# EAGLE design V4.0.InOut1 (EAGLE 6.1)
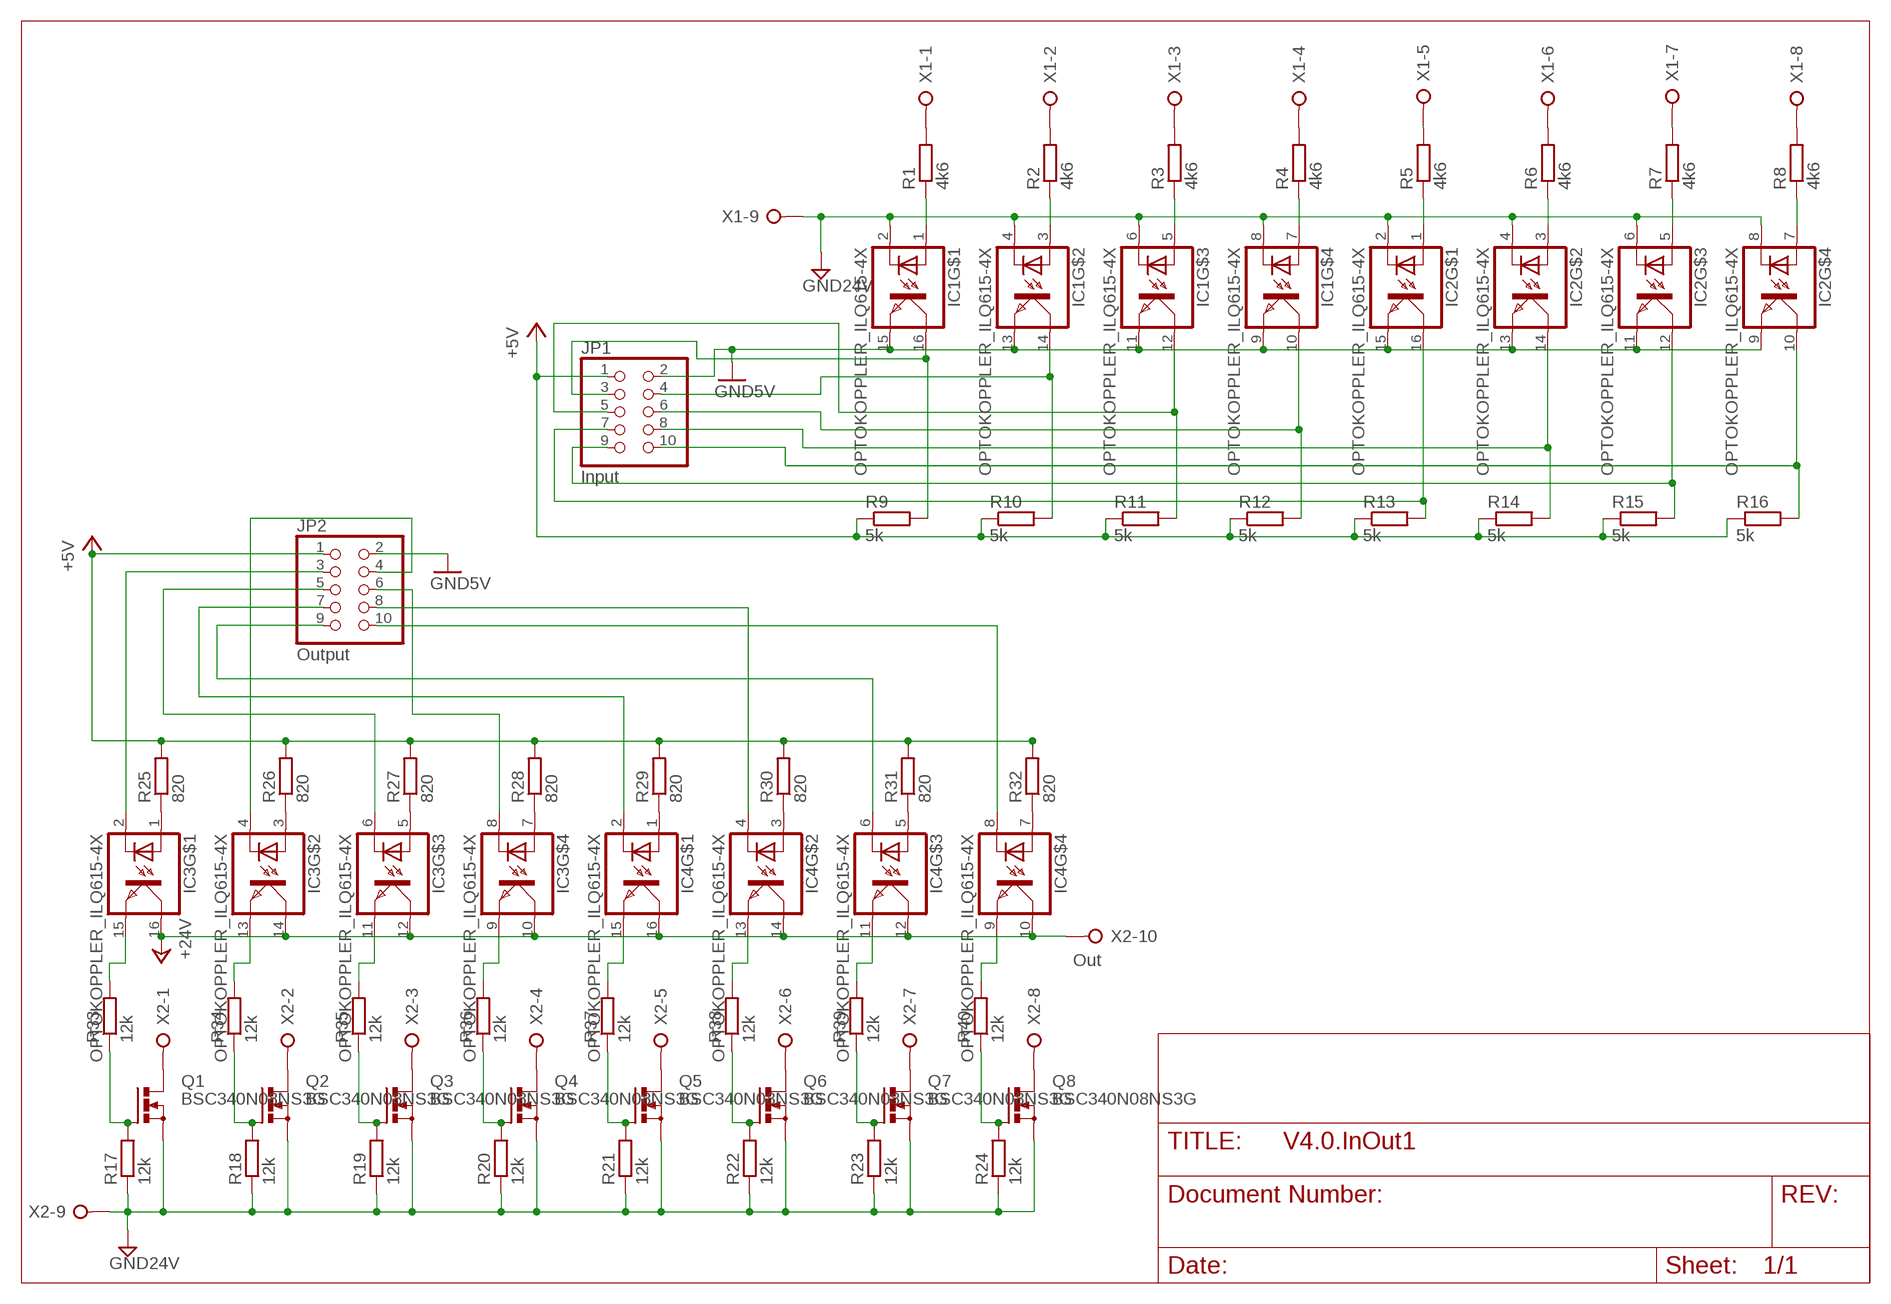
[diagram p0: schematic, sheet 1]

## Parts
IC1  OPTOKOPPLER_ILQ615-4X  [OPTOKOPPLER_ILQ615-4X]
IC2  OPTOKOPPLER_ILQ615-4X  [OPTOKOPPLER_ILQ615-4X]
IC3  OPTOKOPPLER_ILQ615-4X  [OPTOKOPPLER_ILQ615-4X]
IC4  OPTOKOPPLER_ILQ615-4X  [OPTOKOPPLER_ILQ615-4X]
JP1  Input  PINHD-2X5  [2X05]
JP2  Output  PINHD-2X5  [2X05]
Q1  BSC340N08NS3G  [PG-TDSON-8]
Q2  BSC340N08NS3G  [PG-TDSON-8]
Q3  BSC340N08NS3G  [PG-TDSON-8]
Q4  BSC340N08NS3G  [PG-TDSON-8]
Q5  BSC340N08NS3G  [PG-TDSON-8]
Q6  BSC340N08NS3G  [PG-TDSON-8]
Q7  BSC340N08NS3G  [PG-TDSON-8]
Q8  BSC340N08NS3G  [PG-TDSON-8]
R1  4k6  R-EU_R1206  [R1206]
R2  4k6  R-EU_R1206  [R1206]
R3  4k6  R-EU_R1206  [R1206]
R4  4k6  R-EU_R1206  [R1206]
R5  4k6  R-EU_R1206  [R1206]
R6  4k6  R-EU_R1206  [R1206]
R7  4k6  R-EU_R1206  [R1206]
R8  4k6  R-EU_R1206  [R1206]
R9  5k  R-EU_R0402  [R0402]
R10  5k  R-EU_R0402  [R0402]
R11  5k  R-EU_R0402  [R0402]
R12  5k  R-EU_R0402  [R0402]
R13  5k  R-EU_R0402  [R0402]
R14  5k  R-EU_R0402  [R0402]
R15  5k  R-EU_R0402  [R0402]
R16  5k  R-EU_R0402  [R0402]
R17  12k  R-EU_R0402  [R0402]
R18  12k  R-EU_R0402  [R0402]
R19  12k  R-EU_R0402  [R0402]
R20  12k  R-EU_R0402  [R0402]
R21  12k  R-EU_R0402  [R0402]
R22  12k  R-EU_R0402  [R0402]
R23  12k  R-EU_R0402  [R0402]
R24  12k  R-EU_R0402  [R0402]
R25  820  R-EU_R0402  [R0402]
R26  820  R-EU_R0402  [R0402]
R27  820  R-EU_R0402  [R0402]
R28  820  R-EU_R0402  [R0402]
R29  820  R-EU_R0402  [R0402]
R30  820  R-EU_R0402  [R0402]
R31  820  R-EU_R0402  [R0402]
R32  820  R-EU_R0402  [R0402]
R33  12k  R-EU_R0402  [R0402]
R34  12k  R-EU_R0402  [R0402]
R35  12k  R-EU_R0402  [R0402]
R36  12k  R-EU_R0402  [R0402]
R37  12k  R-EU_R0402  [R0402]
R38  12k  R-EU_R0402  [R0402]
R39  12k  R-EU_R0402  [R0402]
R40  12k  R-EU_R0402  [R0402]
X1  In  W237-10P  [W237-10P]
X2  Out  W237-10P  [W237-10P]

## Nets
+5V_IN [+5V]: JP1.1 R9.1 R10.1 R11.1 R12.1 R13.1 R14.1 R15.1 R16.1 ; supply symbol labelled +5V
+5V_OUT [+5V]: JP2.1 R25.2 R26.2 R27.2 R28.2 R29.2 R30.2 R31.2 R32.2 ; supply symbol labelled +5V
+24V: IC3.10(COL) IC3.12(COL) IC3.14(COL) IC3.16(COL) IC4.10(COL) IC4.12(COL) IC4.14(COL) IC4.16(COL) X2.10
AGND_IN [+24V]: IC1.2(C) IC1.4(C) IC1.6(C) IC1.8(C) IC2.2(C) IC2.4(C) IC2.6(C) IC2.8(C) X1.9 ; supply symbol labelled GND24V
AGND_OUT [+24V]: Q1.1(S) Q1.2(S) Q1.3(S) Q2.1(S) Q2.2(S) Q2.3(S) Q3.1(S) Q3.2(S) Q3.3(S) Q4.1(S) Q4.2(S) Q4.3(S) Q5.1(S) Q5.2(S) Q5.3(S) Q6.1(S) Q6.2(S) Q6.3(S) Q7.1(S) Q7.2(S) Q7.3(S) Q8.1(S) Q8.2(S) Q8.3(S) R17.1 R18.1 R19.1 R20.1 R21.1 R22.1 R23.1 R24.1 X2.9 ; supply symbol labelled GND24V
GND [+5V GND]: IC1.9(EMIT) IC1.11(EMIT) IC1.13(EMIT) IC1.15(EMIT) IC2.9(EMIT) IC2.11(EMIT) IC2.13(EMIT) IC2.15(EMIT) JP1.2 JP2.2 ; supply symbol labelled GND5V
N$1: R1.2 X1.1
N$2: R2.2 X1.2
N$3: R3.2 X1.3
N$4: R4.2 X1.4
N$5: R5.2 X1.5
N$6: R6.2 X1.6
N$7: R7.2 X1.7
N$8: R8.2 X1.8
N$9: IC1.16(COL) JP1.3 R9.2
N$10: IC1.1(A) R1.1
N$11: IC1.3(A) R2.1
N$12: IC1.5(A) R3.1
N$13: IC1.7(A) R4.1
N$14: IC2.1(A) R5.1
N$15: IC2.3(A) R6.1
N$16: IC2.5(A) R7.1
N$17: IC2.7(A) R8.1
N$18: IC1.14(COL) JP1.4 R10.2
N$19: IC1.12(COL) JP1.5 R11.2
N$20: IC1.10(COL) JP1.6 R12.2
N$21: IC2.16(COL) JP1.7 R13.2
N$22: IC2.14(COL) JP1.8 R14.2
N$23: IC2.12(COL) JP1.9 R15.2
N$24: IC2.10(COL) JP1.10 R16.2
N$25: Q1.4(G) R17.2 R33.1
N$26: Q2.4(G) R18.2 R34.1
N$27: Q3.4(G) R19.2 R35.1
N$28: Q4.4(G) R20.2 R36.1
N$29: Q5.4(G) R21.2 R37.1
N$30: Q6.4(G) R22.2 R38.1
N$31: Q7.4(G) R23.2 R39.1
N$32: Q8.4(G) R24.2 R40.1
N$33: IC3.3(A) R26.1
N$34: Q1.5(D) Q1.6(D) Q1.7(D) Q1.8(D) X2.1
N$35: IC3.5(A) R27.1
N$36: Q2.5(D) Q2.6(D) Q2.7(D) Q2.8(D) X2.2
N$37: Q3.5(D) Q3.6(D) Q3.7(D) Q3.8(D) X2.3
N$38: Q4.5(D) Q4.6(D) Q4.7(D) Q4.8(D) X2.4
N$39: Q5.5(D) Q5.6(D) Q5.7(D) Q5.8(D) X2.5
N$40: Q6.5(D) Q6.6(D) Q6.7(D) Q6.8(D) X2.6
N$41: Q7.5(D) Q7.6(D) Q7.7(D) Q7.8(D) X2.7
N$42: Q8.5(D) Q8.6(D) Q8.7(D) Q8.8(D) X2.8
N$43: IC3.7(A) R28.1
N$44: IC3.1(A) R25.1
N$45: IC4.1(A) R29.1
N$46: IC4.3(A) R30.1
N$47: IC4.5(A) R31.1
N$48: IC4.7(A) R32.1
N$49: IC3.15(EMIT) R33.2
N$50: IC3.2(C) JP2.3
N$51: IC3.4(C) JP2.4
N$52: IC3.6(C) JP2.5
N$53: IC3.8(C) JP2.6
N$54: IC4.2(C) JP2.7
N$55: IC4.4(C) JP2.8
N$56: IC4.6(C) JP2.9
N$57: IC4.8(C) JP2.10
N$58: IC3.13(EMIT) R34.2
N$59: IC3.11(EMIT) R35.2
N$60: IC3.9(EMIT) R36.2
N$61: IC4.15(EMIT) R37.2
N$62: IC4.13(EMIT) R38.2
N$63: IC4.11(EMIT) R39.2
N$64: IC4.9(EMIT) R40.2
Unconnected: Q1.TH Q2.TH Q3.TH Q4.TH Q5.TH Q6.TH Q7.TH Q8.TH X1.10

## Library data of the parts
IC1-IC4 = Jonas_Bib_Eagle:OPTOKOPPLER_ILQ615-4X: ILQ615-4X009
JP1 JP2 = pinhead:PINHD-2X5: PIN HEADER
Q1-Q8 = transistor-power:BSC340N08NS3G: OptiMOS TM 3 Power-Transistor BSC340N08NS3 G Source: Data sheet
R1-R40 = rcl:R-EU_: RESISTOR, European symbol
X1 X2 = con-wago-508:W237-10P: WAGO SREW CLAMP; OC_FARNELL: unknown; OC_NEWARK: unknown

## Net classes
0 default: width 0.305 mm
1 +5V: width 0.508 mm
2 +5V GND: width 0.508 mm
3 +24V: width 0.508 mm
4 +24V GND: width 0.508 mm

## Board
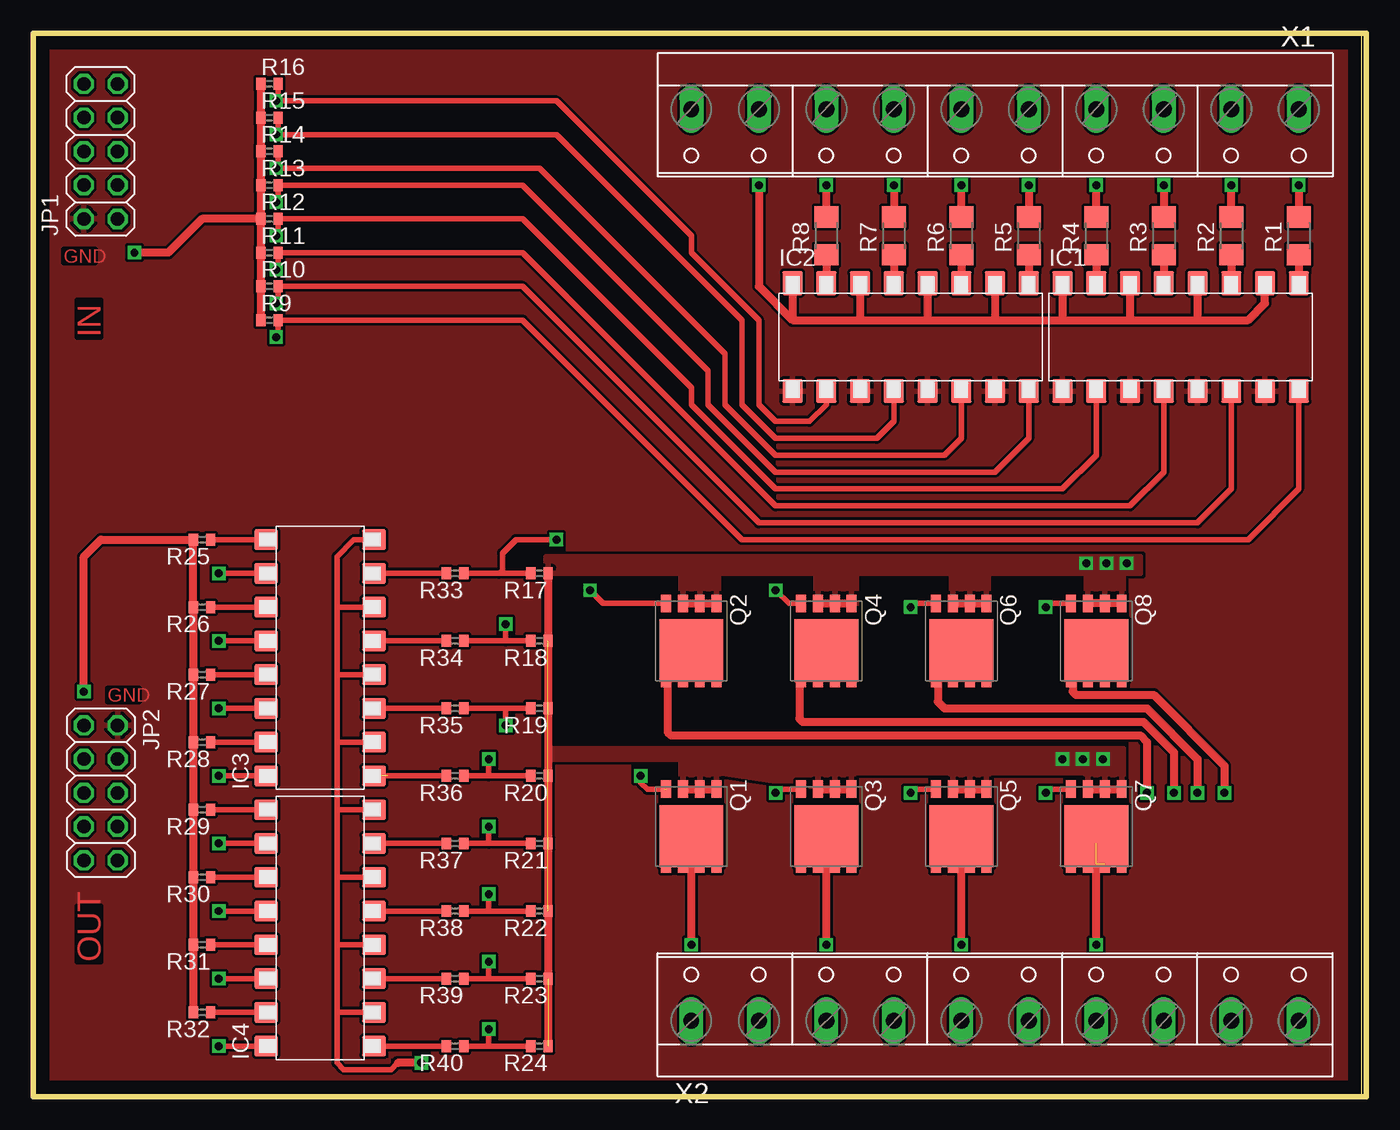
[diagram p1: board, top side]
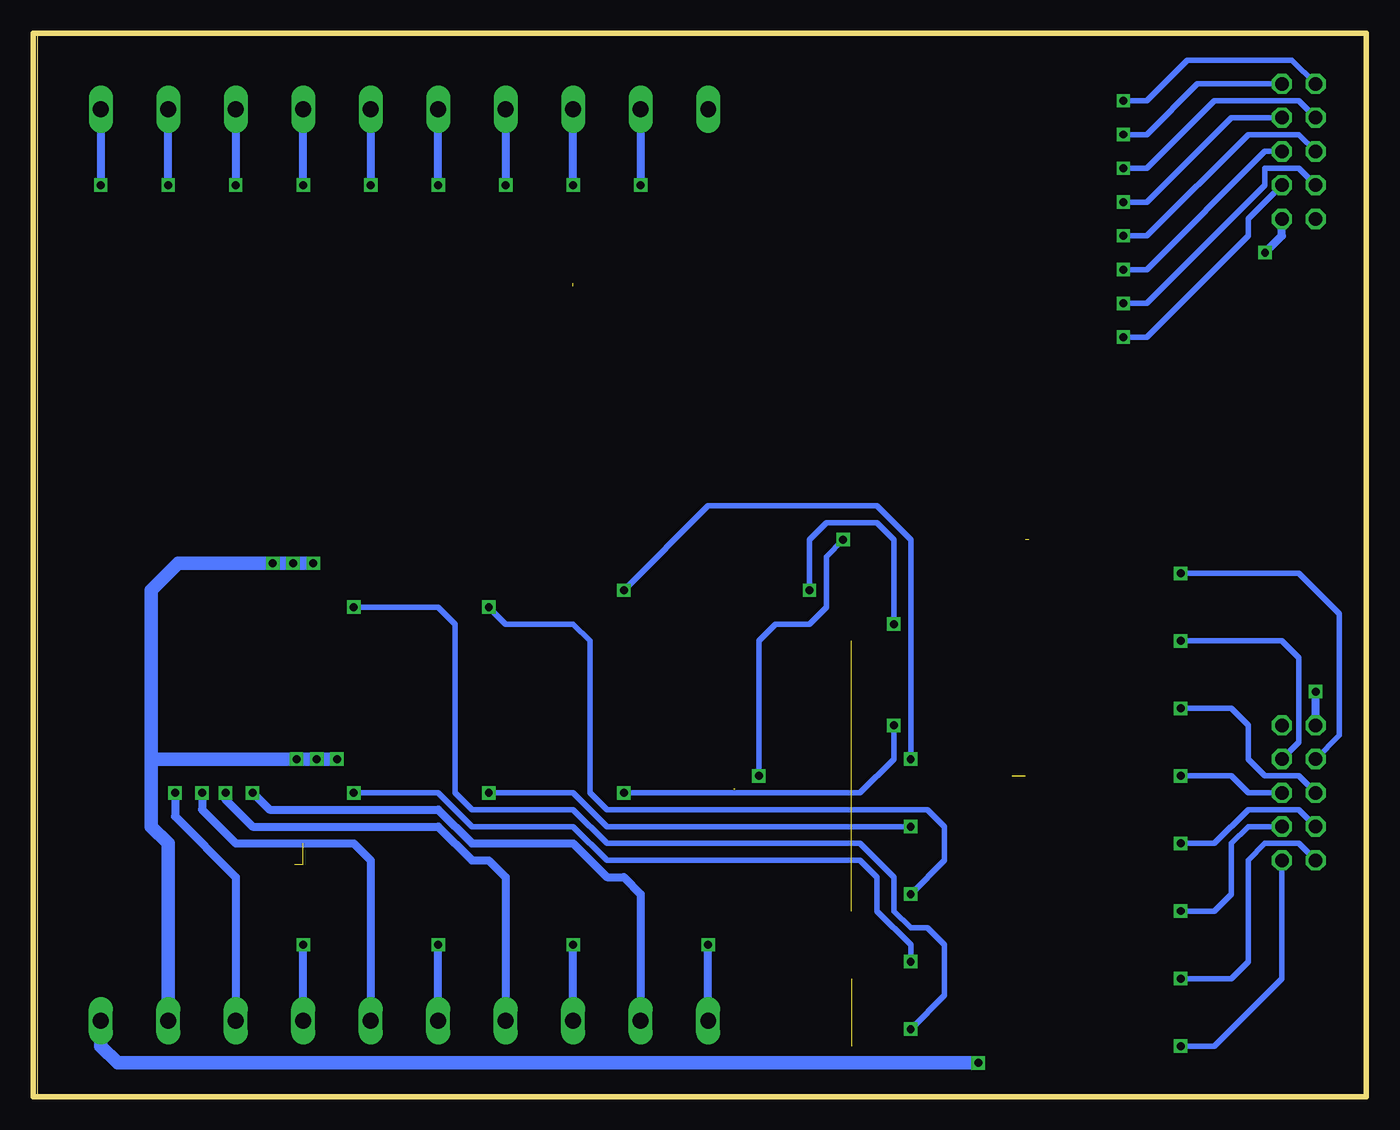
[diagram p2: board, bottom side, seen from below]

Size 100.33 x 80.01 mm. Coordinates in mm from the lower left corner, seen from the top.
Outline: 0,0 100,0 100,80 0,80
Outline: 0,0 100.33,0 100.33,80.01 0,80.01 0,0
Copper layers (1*16): Top 0.035mm / dielectric 1.5mm / Bottom 0.035mm
Design rules: minimum track width 10mil, minimum drill 24mil, track to track 8mil, track to pad 8mil, pad to pad 8mil, via to via 8mil, smd to smd 8mil, copper to edge 40mil, drill to drill 8mil, minimum pad ring 10mil, minimum via ring 8mil, stop-mask expansion 4mil, vias tented up to drill 0mil, thermal gap 10mil

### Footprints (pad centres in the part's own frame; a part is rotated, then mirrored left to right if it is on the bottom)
OPTOKOPPLER_ILQ615-4X = smd 1.525 x 1.78: 1 8.89,4.06; 2 6.35,4.06; 3 3.81,4.06; 4 1.27,4.06; 5 -1.27,4.06; 6 -3.81,4.06; 7 -6.35,4.06; 8 -8.89,4.06; 9 -8.89,-4.06; 10 -6.35,-4.06; 11 -3.81,-4.06; 12 -1.27,-4.06; 13 1.27,-4.06; 14 3.81,-4.06; 15 6.35,-4.06; 16 8.89,-4.06
2X05 = drill 1.016 octagon: 1 -5.08,-1.27; 2 -5.08,1.27; 3 -2.54,-1.27; 4 -2.54,1.27; 5 0,-1.27; 6 0,1.27; 7 2.54,-1.27; 8 2.54,1.27; 9 5.08,-1.27; 10 5.08,1.27
PG-TDSON-8 = smd 1.3 x 0.75: 1 -2.825,1.905; 2 -2.825,0.635; 3 -2.825,-0.635; 4 -2.825,-1.905; 5 2.825,-1.905; 6 2.825,-0.635; 7 2.825,0.635; 8 2.825,1.905 | smd 4.7 x 4.8: TH 0.725,0
R1206 = smd 1.6 x 1.803: 1 -1.422,0; 2 1.422,0
R0402 = smd 0.7 x 0.9: 1 -0.65,0; 2 0.65,0
W237-10P = drill 1.194 long: 1 -22.86,-0.635; 2 -17.78,-0.635; 3 -12.7,-0.635; 4 -7.62,-0.635; 5 -2.54,-0.635; 6 2.54,-0.635; 7 7.62,-0.635; 8 12.7,-0.635; 9 17.78,-0.635; 10 22.86,-0.635

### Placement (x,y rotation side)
IC1  86.36,57.15 0 top
IC2  66.04,57.15 0 top
IC3  21.59,33.02 90 top
IC4  21.59,12.7 90 top
JP1  5.08,71.12 90 top
JP2  5.08,22.86 270 top
Q1  49.53,20.32 270 top
Q2  49.53,34.29 270 top
Q3  59.69,20.32 270 top
Q4  59.69,34.29 270 top
Q5  69.85,20.32 270 top
Q6  69.85,34.29 270 top
Q7  80.01,20.32 270 top
Q8  80.01,34.29 270 top
R1  95.25,64.77 90 top
R2  90.17,64.77 90 top
R3  85.09,64.77 90 top
R4  80.01,64.77 90 top
R5  74.93,64.77 90 top
R6  69.85,64.77 90 top
R7  64.77,64.77 90 top
R8  59.69,64.77 90 top
R9  17.78,58.42 0 top
R10  17.78,60.96 0 top
R11  17.78,63.5 0 top
R12  17.78,66.04 0 top
R13  17.78,68.58 0 top
R14  17.78,71.12 0 top
R15  17.78,73.66 0 top
R16  17.78,76.2 0 top
R17  38.1,39.37 180 top
R18  38.1,34.29 180 top
R19  38.1,29.21 180 top
R20  38.1,24.13 180 top
R21  38.1,19.05 180 top
R22  38.1,13.97 180 top
R23  38.1,8.89 180 top
R24  38.1,3.81 180 top
R25  12.7,41.91 180 top
R26  12.7,36.83 180 top
R27  12.7,31.75 180 top
R28  12.7,26.67 180 top
R29  12.7,21.59 180 top
R30  12.7,16.51 180 top
R31  12.7,11.43 180 top
R32  12.7,6.35 180 top
R33  31.75,39.37 180 top
R34  31.75,34.29 180 top
R35  31.75,29.21 180 top
R36  31.75,24.13 180 top
R37  31.75,19.05 180 top
R38  31.75,13.97 180 top
R39  31.75,8.89 180 top
R40  31.75,3.81 180 top
X1  72.39,73.66 180 top
X2  72.39,6.35 0 top

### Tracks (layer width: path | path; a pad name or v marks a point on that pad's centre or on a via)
+5V_IN  (via drill 0.6)
  Top 0.61: R12.1 12.7,66.04 10.16,63.5 v7.62,63.5 | R16.1 R15.1 R14.1 R13.1 R12.1 | R12.1 R11.1 R10.1 R9.1
  Bottom 0.61: v7.62,63.5 6.35,64.77 JP1.1
+5V_OUT  (via drill 0.6)
  Top 0.61: v3.81,30.48 3.81,40.64 5.08,41.91 R25.2 R26.2 R27.2 R28.2 R29.2 R30.2 R31.2 R32.2
  Bottom 0.61: JP2.1 v3.81,30.48
+24V  (via drill 0.6)  (1 unrouted)
  Top 0.406: 27.43,2.54 26.92,2.03 23.37,2.03 22.86,2.54 22.86,6.35 | 22.86,6.35 22.86,11.43 | 22.86,11.43 22.86,16.51 | 22.86,16.51 22.86,21.59 | 22.86,21.59 22.86,26.67 | 22.86,26.67 22.86,31.75 | 22.86,31.75 22.86,36.83 | 22.86,36.83 22.86,40.64 24.13,41.91 25.4,41.91 | IC3.14 22.86,36.83 | IC3.12 22.86,31.75 | IC3.10 22.86,26.67 | IC4.10 22.86,6.35 | IC4.12 22.86,11.43 | IC4.14 22.86,16.51 | IC4.16 22.86,21.59
  Top 0.61: v29.21,2.54 27.43,2.54
  Bottom 1.016: X2.10 95.25,3.81 93.98,2.54 v29.21,2.54
AGND_IN  (via drill 0.6)
  Top 0.61: v54.61,68.58 54.61,60.96 57.15,58.42 | 57.15,58.42 62.23,58.42 | 62.23,58.42 67.31,58.42 | 67.31,58.42 72.39,58.42 | 72.39,58.42 77.47,58.42 | 77.47,58.42 82.55,58.42 | 82.55,58.42 87.63,58.42 | 87.63,58.42 91.44,58.42 92.71,59.69 IC1.2 | IC2.8 57.15,58.42 | IC2.6 62.23,58.42 | IC2.4 67.31,58.42 | IC2.2 72.39,58.42 | IC1.8 77.47,58.42 | IC1.6 82.55,58.42 | IC1.4 87.63,58.42
  Bottom 0.61: X1.9 v54.61,68.58
AGND_OUT  (via drill 0.6)  (6 unrouted)
  Top 0.406: 79.53,37.12 79.5,37.08
  Top 0.61: R20.1 R24.1 | Q2.3 Q2.1 | Q4.3 Q4.1 | Q6.3 Q6.1 | Q1.3 51.28,23.14 | Q3.3 Q3.1 | Q5.3 Q5.1 | Q7.3 Q7.1 | Q8.1 79.53,37.12 | R17.1 38.75,24.24
  Bottom 1.016: X2.9 90.17,19.05 91.44,20.32 91.44,25.4 | 91.44,25.4 91.44,38.1 89.41,40.13 v82.3,40.13 v80.77,40.13 v79.25,40.13 | 91.44,25.4 v80.52,25.4 v78.99,25.4 v77.47,25.4
  pour Top: 82.55,40.64 38.61,40.64 38.61,39.37 48.77,39.37 48.77,36.83 51.56,36.83 51.56,38.86 51.56,39.37 58.93,39.37 58.93,36.83 61.98,36.83 61.98,39.37 69.09,39.37 69.09,37.08 71.88,37.08 71.88,39.37 79.25,39.37 79.25,36.83 82.04,36.83 82.04,39.37 82.55,39.37 83.31,39.37 83.31,40.64
  pour Top: 38.86,25.4 48.77,25.4 48.77,22.86 51.56,22.86 51.56,24.38 61.72,22.86 61.72,24.38 69.09,24.38 69.09,22.86 71.88,22.86 71.88,24.38 79.25,24.38 79.25,22.86 82.04,22.86 82.04,26.16 38.86,26.16
GND
  pour Top (rank 2): 0,80.01 0,0 100.33,0 100.33,80.01
N$1  (via drill 0.6)
  Top 0.61: v95.25,68.58 R1.2
  Bottom 0.61: X1.1 v95.25,68.58
N$2  (via drill 0.6)
  Top 0.61: R2.2 v90.17,68.58
  Bottom 0.61: v90.17,68.58 X1.2
N$3  (via drill 0.6)
  Top 0.61: v85.09,68.58 R3.2
  Bottom 0.61: X1.3 v85.09,68.58
N$4  (via drill 0.6)
  Top 0.61: R4.2 v80.01,68.58
  Bottom 0.61: v80.01,68.58 X1.4
N$5  (via drill 0.6)
  Top 0.61: v74.93,68.58 R5.2
  Bottom 0.61: X1.5 v74.93,68.58
N$6  (via drill 0.6)
  Top 0.61: R6.2 v69.85,68.58
  Bottom 0.61: v69.85,68.58 X1.6
N$7  (via drill 0.6)
  Top 0.61: v64.77,68.58 R7.2
  Bottom 0.61: X1.7 v64.77,68.58
N$8  (via drill 0.6)
  Top 0.61: R8.2 v59.69,68.58
  Bottom 0.61: v59.69,68.58 X1.8
N$9  (via drill 0.6)
  Top 0.406: IC1.16 95.25,45.72 91.44,41.91 53.34,41.91 36.83,58.42 R9.2 18.43,57.29 v18.29,57.15
  Bottom 0.406: v18.29,57.15 16.51,57.15 8.89,64.77 8.89,66.04 JP1.3
N$10
  Top 0.61: R1.1 IC1.1
N$11
  Top 0.61: R2.1 IC1.3
N$12
  Top 0.61: R3.1 IC1.5
N$13
  Top 0.61: R4.1 IC1.7
N$14
  Top 0.61: R5.1 IC2.1
N$15
  Top 0.61: R6.1 IC2.3
N$16
  Top 0.61: R7.1 IC2.5
N$17  (1 unrouted)
  Top 0.61: R8.1 59.69,60.96
N$18  (via drill 0.6)
  Top 0.406: IC1.14 90.17,45.72 87.63,43.18 54.61,43.18 36.83,60.96 R10.2 18.43,59.83 v18.29,59.69
  Bottom 0.406: v18.29,59.69 16.51,59.69 7.62,68.58 7.62,69.85 5.08,69.85 JP1.4
N$19  (via drill 0.6)
  Top 0.406: IC1.12 85.09,46.99 82.55,44.45 55.88,44.45 36.83,63.5 R11.2 18.43,62.37 v18.29,62.23
  Bottom 0.406: v18.29,62.23 16.51,62.23 7.62,71.12 JP1.5
N$20  (via drill 0.6)
  Top 0.406: IC1.10 80.01,48.26 77.47,45.72 55.88,45.72 49.53,52.07 49.53,53.34 36.83,66.04 R12.2 18.43,64.91 v18.29,64.77
  Bottom 0.406: v18.29,64.77 16.51,64.77 8.89,72.39 5.08,72.39 JP1.6
N$21  (via drill 0.6)
  Top 0.406: IC2.16 74.93,49.53 72.39,46.99 55.88,46.99 50.8,52.07 50.8,54.61 36.83,68.58 R13.2 18.43,67.45 v18.29,67.31
  Bottom 0.406: v18.29,67.31 16.51,67.31 10.16,73.66 JP1.7
N$22  (via drill 0.6)
  Top 0.406: R14.2 18.43,69.99 v18.29,69.85 38.1,69.85 52.07,55.88 52.07,52.07 55.88,48.26 68.58,48.26 69.85,49.53 IC2.14
  Bottom 0.406: v18.29,69.85 16.51,69.85 11.43,74.93 5.08,74.93 JP1.8
N$23  (via drill 0.6)
  Top 0.406: R15.2 18.43,72.53 v18.29,72.39 39.37,72.39 53.34,58.42 53.34,52.07 55.88,49.53 63.5,49.53 64.77,50.8 IC2.12
  Bottom 0.406: v18.29,72.39 16.51,72.39 12.7,76.2 JP1.9
N$24  (via drill 0.6)
  Top 0.406: R16.2 18.43,75.07 v18.29,74.93 39.37,74.93 49.53,64.77 49.53,63.5 54.61,58.42 54.61,52.07 55.88,50.8 58.42,50.8 59.69,52.07 IC2.10
  Bottom 0.406: v18.29,74.93 16.51,74.93 13.46,77.98 5.59,77.98 JP1.10
N$25  (via drill 0.6)  (1 unrouted)
  Top 0.406: R17.2 35.05,39.37 | 35.05,39.37 R33.1 | v39.37,41.91 36.32,41.91 35.31,40.89 35.31,39.62 35.05,39.37 | v45.72,24.13 45.72,23.62 46.23,23.11 47.5,23.11
  Bottom 0.406: v39.37,41.91 40.64,40.64 40.64,36.83 41.91,35.56 44.45,35.56 45.72,34.29 v45.72,24.13
N$26  (via drill 0.6)
  Top 0.406: R18.2 35.56,34.29 | 35.56,34.29 R34.1 | Q2.4 42.9,37.12 v41.91,38.1 | v35.56,35.56 35.56,34.29
  Bottom 0.406: v41.91,38.1 41.91,41.91 40.64,43.18 36.83,43.18 35.56,41.91 v35.56,35.56
N$27  (via drill 0.6)
  Top 0.406: R19.2 35.56,29.21 | 35.56,29.21 R35.1 | Q3.4 56.16,23.14 v55.88,22.86 | v35.56,27.94 35.56,29.21
  Bottom 0.406: v55.88,22.86 38.1,22.86 35.56,25.4 v35.56,27.94
N$28  (via drill 0.6)
  Top 0.406: R20.2 34.29,24.13 | 34.29,24.13 R36.1 | Q4.4 56.87,37.12 v55.88,38.1 | v34.29,25.4 34.29,24.13
  Bottom 0.406: v55.88,38.1 49.53,44.45 36.83,44.45 34.29,41.91 v34.29,25.4
N$29  (via drill 0.6)
  Top 0.406: R21.2 34.29,19.05 | 34.29,19.05 R37.1 | Q5.4 66.33,23.14 v66.04,22.86 | v34.29,20.32 34.29,19.05
  Bottom 0.406: v66.04,22.86 59.69,22.86 57.15,20.32 v34.29,20.32
N$30  (via drill 0.6)
  Top 0.406: R22.2 34.29,13.97 | 34.29,13.97 R38.1 | Q6.4 66.33,37.12 v66.04,36.83 | v34.29,15.24 34.29,13.97
  Bottom 0.406: v66.04,36.83 64.77,35.56 59.69,35.56 58.42,34.29 58.42,22.86 57.15,21.59 33.02,21.59 31.75,20.32 31.75,17.78 v34.29,15.24
N$31  (via drill 0.6)
  Top 0.406: R23.2 34.29,8.89 | 34.29,8.89 R39.1 | Q7.4 76.48,23.14 v76.2,22.86 | v34.29,10.16 34.29,8.89
  Bottom 0.406: v76.2,22.86 69.85,22.86 67.31,20.32 59.69,20.32 57.15,17.78 38.1,17.78 36.83,16.51 36.83,13.97 34.29,11.43 v34.29,10.16
N$32  (via drill 0.6)
  Top 0.406: R24.2 34.29,3.81 | 34.29,3.81 R40.1 | Q8.4 76.48,37.12 v76.2,36.83 | v34.29,5.08 34.29,3.81
  Bottom 0.406: v76.2,36.83 69.85,36.83 68.58,35.56 68.58,22.86 67.31,21.59 59.69,21.59 57.15,19.05 38.1,19.05 35.56,16.51 35.56,13.97 34.29,12.7 33.02,12.7 31.75,11.43 31.75,7.62 v34.29,5.08
N$33
  Top 0.406: R26.1 IC3.3
N$34  (via drill 0.6)
  Top 0.61: v49.53,11.43 49.53,17.5 | 49.53,19.05 49.53,17.78 49.53,17.5 | Q1.7 49.53,17.5
  Bottom 0.61: X2.1 v49.53,11.43
N$35
  Top 0.406: R27.1 IC3.5
N$36  (via drill 0.6)
  Top 0.406: Q2.8 47.98,31.46 47.75,31.24
  Top 0.61: 47.75,31.24 47.75,27.43 48.01,27.18 83.31,27.18 83.82,26.67 v83.82,22.86
  Bottom 0.61: v83.82,22.86 82.55,21.59 69.85,21.59 67.31,19.05 59.69,19.05 57.15,16.51 55.88,16.51 54.61,15.24 X2.2
N$37  (via drill 0.6)
  Top 0.61: v59.69,11.43 59.69,17.5 | 59.69,19.05 59.69,17.78 59.69,17.5 | Q3.7 59.69,17.5
  Bottom 0.61: X2.3 v59.69,11.43
N$38  (via drill 0.6)
  Top 0.406: Q4.8 57.88,31.46 57.66,31.24
  Top 0.61: 57.66,31.24 57.66,28.45 57.91,28.19 83.57,28.19 85.85,25.91 v85.85,22.86
  Bottom 0.406: v85.85,22.86 85.85,22.35
  Bottom 0.61: 85.85,22.35 83.82,20.32 69.85,20.32 67.31,17.78 66.04,17.78 64.77,16.51 X2.4
N$39  (via drill 0.6)
  Top 0.61: v69.85,11.43 69.85,17.5 | 69.85,19.05 69.85,17.78 69.85,17.5 | Q5.7 69.85,17.5
  Bottom 0.61: X2.5 v69.85,11.43
N$40  (via drill 0.6)
  Top 0.406: Q6.8 68.3,31.46 68.07,31.24
  Top 0.61: 68.07,31.24 68.07,29.72 68.58,29.21 83.82,29.21 87.63,25.4 v87.63,22.86
  Bottom 0.61: v87.63,22.86 87.63,21.59 85.09,19.05 76.2,19.05 74.93,17.78 X2.6
N$41  (via drill 0.6)  (3 unrouted)
  Top 0.61: v80.01,11.43 80.01,17.5
  Bottom 0.61: X2.7 v80.01,11.43
N$42  (via drill 0.6)
  Top 0.406: Q8.8 78.45,31.46 78.23,31.24
  Top 0.61: 78.23,31.24 78.23,30.48 78.49,30.23 84.33,30.23 89.66,24.89 v89.66,22.86
  Bottom 0.61: v89.66,22.86 89.66,21.08 85.09,16.51 X2.8
N$43
  Top 0.406: IC3.7 R28.1
N$44
  Top 0.406: R25.1 IC3.1
N$45
  Top 0.406: IC4.1 R29.1
N$46
  Top 0.406: IC4.3 R30.1
N$47
  Top 0.406: IC4.5 R31.1
N$48
  Top 0.406: IC4.7 R32.1
N$49
  Top 0.406: R33.2 IC3.15
N$50  (via drill 0.6)
  Top 0.406: IC3.2 v13.97,39.37
  Bottom 0.406: v13.97,39.37 5.08,39.37 2.03,36.32 2.03,27.18 JP2.3
N$51  (via drill 0.6)
  Top 0.406: IC3.4 v13.97,34.29
  Bottom 0.406: v13.97,34.29 6.35,34.29 5.08,33.02 5.08,26.67 JP2.4
N$52  (via drill 0.6)
  Top 0.406: IC3.6 v13.97,29.21
  Bottom 0.406: v13.97,29.21 10.16,29.21 8.89,27.94 8.89,25.4 7.62,24.13 5.08,24.13 JP2.5
N$53  (via drill 0.6)
  Top 0.406: IC3.8 v13.97,24.13
  Bottom 0.406: v13.97,24.13 10.16,24.13 8.89,22.86 JP2.6
N$54  (via drill 0.6)
  Top 0.406: IC4.2 v13.97,19.05
  Bottom 0.406: v13.97,19.05 11.43,19.05 8.89,21.59 5.08,21.59 JP2.7
N$55  (via drill 0.6)
  Top 0.406: IC4.4 v13.97,13.97
  Bottom 0.406: v13.97,13.97 11.43,13.97 10.16,15.24 10.16,19.05 8.89,20.32 JP2.8
N$56  (via drill 0.6)
  Top 0.406: IC4.6 v13.97,8.89
  Bottom 0.406: v13.97,8.89 10.16,8.89 8.89,10.16 8.89,17.78 7.62,19.05 5.08,19.05 JP2.9
N$57  (via drill 0.6)
  Top 0.406: IC4.8 v13.97,3.81
  Bottom 0.406: v13.97,3.81 11.43,3.81 6.35,8.89 JP2.10
N$58
  Top 0.406: R34.2 IC3.13
N$59
  Top 0.406: R35.2 IC3.11
N$60  (1 unrouted)
  Top 0.406: R36.2 26.67,24.13
N$61
  Top 0.406: R37.2 IC4.15
N$62
  Top 0.406: R38.2 IC4.13
N$63
  Top 0.406: R39.2 IC4.11
N$64
  Top 0.406: R40.2 IC4.9

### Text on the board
Top: GND | IN | GND | OUT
